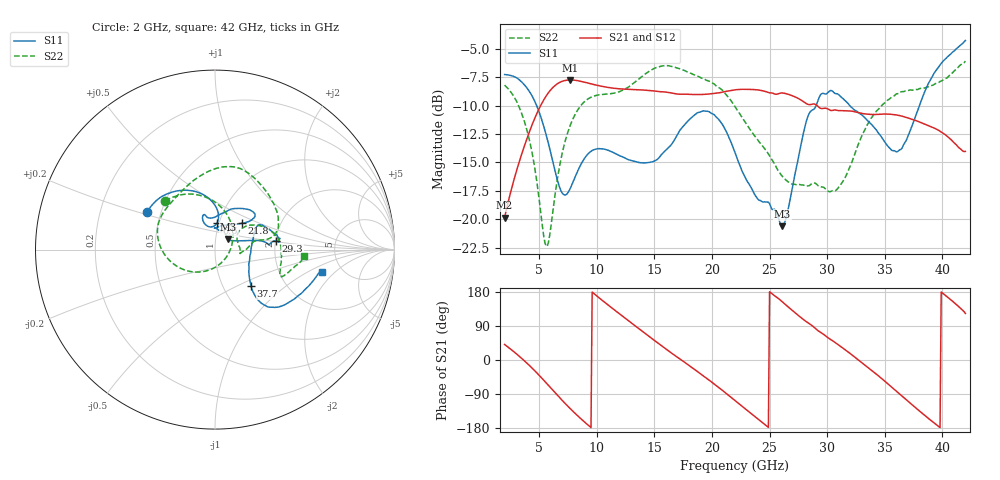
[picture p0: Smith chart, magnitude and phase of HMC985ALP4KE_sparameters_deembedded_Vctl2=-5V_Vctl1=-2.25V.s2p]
!s2p File: Measurements: S11, S21, S12, S22
# GHz S dB R 50.0
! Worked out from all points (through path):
!   401 points, 2 GHz to 42 GHz, reference 50 ohm
!   highest |S21| = -7.75 dB at 7.7 GHz (marker M1); lowest = -19.9 dB at 2 GHz (marker M2)
!   lowest |S11| = -20.6 dB at 26.1 GHz (marker M3), VSWR 1.21, Z = 57.5 + j6.71 ohm
!   |S11| at or under -10 dB: 4.777 GHz to 29.04 GHz (24.26 GHz wide, 144 % of centre); 31.95 GHz to 38 GHz (6.049 GHz wide, 17.3 % of centre)
!   |S22| runs from -22.4 to -6.1 dB; largest |S21 - S12| = 0.0005
!   S11 on the Smith chart (normalised r, x): 2 GHz: 0.42, +0.21; 6.6 GHz: 0.98, +0.29; 21.8 GHz: 1.28, +0.39; 29.3 GHz: 2.01, +0.22; 37.7 GHz: 1.35, -0.60; 42 GHz: 3.54, -1.40
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2  -7.27 151.1  -19.85 41.0  -19.86 41.0  -8.21 135.7
4  -8.54 117.9  -12.73 -10.0  -12.74 -10.0  -12.40 82.1
5.6  -12.56 88.4  -9.17 -60.1  -9.18 -60.1  -22.37 -29.5
6.6  -16.62 85.9  -8.07 -93.5  -8.08 -93.5  -16.34 -124.9
7.7  -17.29 107.4  -7.75 -128.5  -7.76 -128.5  -11.73 -166.1
8.7  -15.04 112.5  -7.89 -157.2  -7.89 -157.2  -9.90 170.8
10.3  -13.80 107.5  -8.28 161.7  -8.29 161.7  -9.05 147.4
12.3  -14.54 104.0  -8.55 114.2  -8.56 114.2  -8.63 122.5
15.4  -14.60 87.2  -8.78 42.7  -8.79 42.7  -6.59 81.0
18.4  -10.91 52.4  -9.03 -23.0  -9.03 -23.0  -7.28 49.3
21.8  -13.61 44.6  -8.65 -102.0  -8.65 -102.0  -9.79 12.3
22  -14.13 47.1  -8.62 -107.0  -8.62 -107.0  -10.09 11.7
24.1  -18.33 88.2  -8.64 -158.3  -8.65 -158.3  -13.21 11.3
26.1  -20.61 38.4  -8.90 153.7  -8.90 153.7  -16.21 -3.9
28.7  -10.40 4.9  -9.88 90.5  -9.89 90.5  -16.83 -3.8
29.3  -9.30 8.3  -10.17 75.4  -10.17 75.4  -17.11 0.1
30.9  -8.98 12.8  -10.43 41.3  -10.44 41.3  -17.32 25.6
32.4  -10.42 25.7  -10.55 7.6  -10.55 7.6  -14.28 38.3
35.4  -13.71 6.7  -10.76 -66.3  -10.76 -66.3  -9.44 15.8
37.7  -10.88 -45.4  -11.32 -126.5  -11.32 -126.5  -8.58 -6.3
39.7  -6.55 -43.1  -12.19 -175.9  -12.20 -175.9  -7.97 -22.3
42  -4.28 -11.7  -14.03 122.7  -14.03 122.8  -6.09 -3.9
